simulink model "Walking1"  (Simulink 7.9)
settings: Solver=ode45  StartTime=0.0  StopTime=10.0  RelTol=1e-3
InitFcn:
  | dt0=0.01;
libraries: arduinolib x9

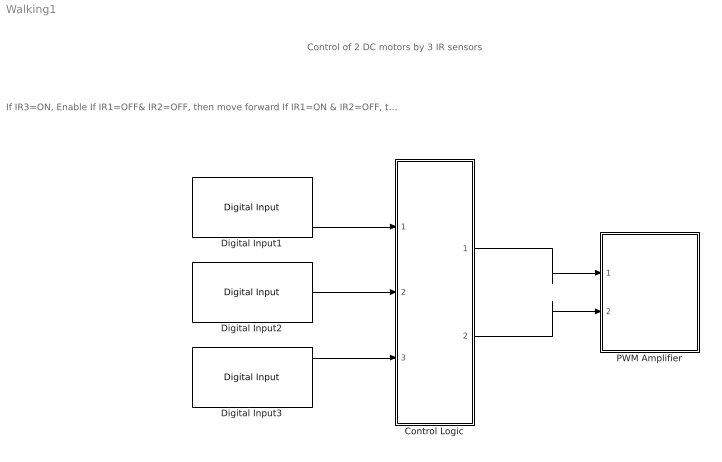
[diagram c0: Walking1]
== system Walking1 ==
  note: Control of 2 DC motors by 3 IR sensors
  note: If IR3=ON, Enable If IR1=OFF& IR2=OFF, then move forward If IR1=ON & IR2=OFF, then turn left If IR1=OFF & IR2=ON, then turn right If IR1=ON & IR2=ON, then move backward
  Control Logic : MATLAB Function  TreatAsAtomicUnit=on
  Digital Input1 : arduinolib/Digital Input  pinNumber=26  sampleTime=dt0
  Digital Input2 : arduinolib/Digital Input  pinNumber=27  sampleTime=dt0
  Digital Input3 : arduinolib/Digital Input  pinNumber=28  sampleTime=dt0
  PWM Amplifier : Subsystem  TreatAsAtomicUnit=on
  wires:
  Digital Input1/1 -> Control Logic/1(u1)
  Digital Input2/1 -> Control Logic/2(u2)
  Control Logic/1(out1) -> PWM Amplifier/1(In1)
  Control Logic/2(out2) -> PWM Amplifier/2(In2)
  Digital Input3/1 -> Control Logic/3(u3)

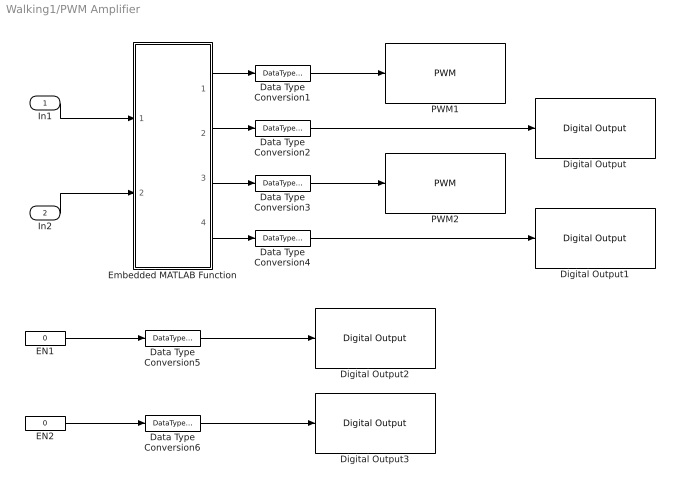
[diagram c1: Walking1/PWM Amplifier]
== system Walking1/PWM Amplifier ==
  In1 : Inport
  In2 : Inport  Port=2
  Data Type Conversion{1..6} (6 alike) : DataTypeConversion  OutDataTypeStr=uint8
  Digital Output : arduinolib/Digital Output  pinNumber=24
  Digital Output1 : arduinolib/Digital Output  pinNumber=25
  Digital Output2 : arduinolib/Digital Output  pinNumber=22
  Digital Output3 : arduinolib/Digital Output  pinNumber=23
  EN1 : Constant  Value=0
  EN2 : Constant  Value=0
  Embedded MATLAB Function : MATLAB Function  TreatAsAtomicUnit=on
  PWM1 : arduinolib/PWM  pinNumber=2
  PWM2 : arduinolib/PWM  pinNumber=3
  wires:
  In1/1 -> Embedded MATLAB Function/1(u1)
  In2/1 -> Embedded MATLAB Function/2(u2)
  Embedded MATLAB Function/1(pwm1) -> Data Type Conversion1/1
  Embedded MATLAB Function/3(pwm2) -> Data Type Conversion3/1
  Embedded MATLAB Function/2(dir1) -> Data Type Conversion2/1
  Embedded MATLAB Function/4(dir2) -> Data Type Conversion4/1
  EN1/1 -> Data Type Conversion5/1
  EN2/1 -> Data Type Conversion6/1
  Data Type Conversion1/1 -> PWM1/1
  Data Type Conversion2/1 -> Digital Output/1
  Data Type Conversion3/1 -> PWM2/1
  Data Type Conversion4/1 -> Digital Output1/1
  Data Type Conversion5/1 -> Digital Output2/1
  Data Type Conversion6/1 -> Digital Output3/1

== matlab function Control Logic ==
function [out1, out2] = fcn(u1, u2, u3)

% When IR sensor is blocked (or reflected), u=0
% When IR sensor is not blocked (or not reflected), u=1
out1=0; out2=0;
%sp1=250; sp2=-250; 
sp1=-190; sp2=150;      % 0~255 %
if u3==0,
    if u1==1 && u2==1,  out1=sp1; out2=sp2; end     % Forward %
    if u1==0 && u2==1,  out1=0; out2=sp2; end     % Left %
    if u1==1 && u2==0,  out1=sp1; out2=0; end     % Right %
    if u1==0 && u2==0,  out1=-sp1; out2=-sp2; end     % Backward %
else
    out1=0; out2=0;
end

== matlab function PWM Amplifier/Embedded
MATLAB Function ==
function [pwm1, dir1, pwm2, dir2] = fcn(u1, u2)

if u1>=0,dir1=1;
else dir1=0; end

if u2>=0,dir2=1;    
else dir2=0; end

pwm1=abs(u1);
pwm2=abs(u2);
% Saturation %
if pwm1>=255, pwm1=255; end
if pwm2>=255, pwm2=255; end
